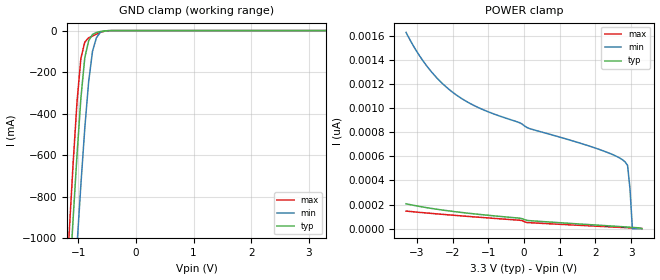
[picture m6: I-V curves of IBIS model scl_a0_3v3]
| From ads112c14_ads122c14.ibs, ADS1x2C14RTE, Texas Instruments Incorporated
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|   Model scl_a0_3v3
[Model] scl_a0_3v3
Model_type Input
Polarity   Non-Inverting
Enable   Active-High
Vinl =  0.990V
Vinh =  2.310V
C_comp   1.000pF   0.500pF   2.000pF
[Model Spec]
Vinh   2.310V   2.100V   2.520V
Vinl   0.990V   0.900V   1.080V
[Temperature Range]   27.000   0.125k   -40.000
[Voltage Range]   3.300V   3.000V   3.600V
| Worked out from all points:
|   GND clamp passes 1 mA (typ) near -0.51 V on its own axis
[GND_clamp]
|Voltage   I(typ)   I(min)   I(max)
-3.3V     -8.28A     -7.976A    -8.613A
-1.156V   -1.224A    -1.66A     -963mA
-1.089V   -901.1mA   -1.342A    -635.5mA
-1.022V   -595.6mA   -1.034A    -340.6mA
-955mV    -324.7mA   -739.9mA   -133.8mA
-888mV    -131.2mA   -471mA     -55.55mA
-821mV    -49.34mA   -247.1mA   -34.58mA
-754mV    -18.25mA   -99.81mA   -26.62mA
-687mV    -9.129mA   -35.22mA   -17.27mA
-620mV    -4.609mA   -8.672mA   -8.764mA
-553mV    -1.974mA   -1.956mA   -3.638mA
3.3V      0A         0A         0A
[POWER_clamp]
|Voltage   I(typ)   I(min)   I(max)
-3.3V     206.4pA    1.628nA    145.8pA
-2.931V   184.9pA    1.438nA    135.4pA
-2.529V   165.2pA    1.28nA     124.9pA
-2.127V   148.3pA    1.163nA    114.9pA
-1.658V   131.3pA    1.064nA    103.8pA
151mV     66.54pA    830.8pA    49.54pA
1.96V     31pA       672.2pA    21.53pA
2.764V    15.84pA    569.7pA    9.562pA
2.898V    13.25pA    524.8pA    7.587pA
2.965V    11.94pA    331.4pA    6.602pA
3.032V    10.6pA     0A         5.618pA
3.3V      0A         0A         1.691pA
